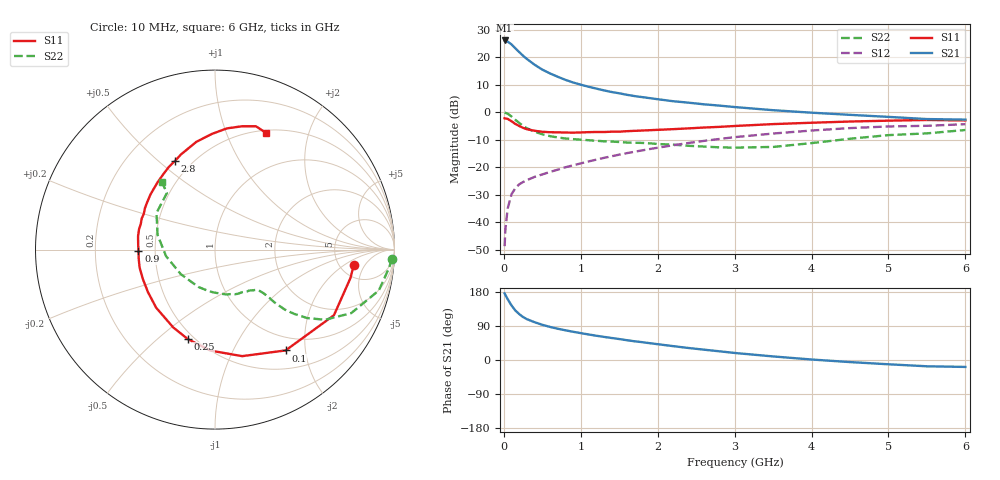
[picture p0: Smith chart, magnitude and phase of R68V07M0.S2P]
! SIEMENS Small Signal Semiconductors
! BFR193
! Si NPN RF Bipolar Junction Transistor in SOT23
! VCE = 8 V  IC = 7 mA
! Common Emitter S-Parameters:  May  1996
# GHz  S  MA  R  50
!  f  S11  S21  S12  S22
! GHz  MAG  ANG  MAG  ANG  MAG  ANG  MAG  ANG
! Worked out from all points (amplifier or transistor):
!   36 points, 10 MHz to 6 GHz, reference 50 ohm
!   highest |S21| = 26.1 dB at 10 MHz (marker M1)
!   |S21| within 3 dB of that: start of sweep to 154.8 MHz
!   unconditionally stable (mu >= 1): 840.8 MHz to 2.029 GHz
!   at 250 MHz: K = 0.52, MSG = 22.9 dB, |S12| = -25.3 dB
!   at 1.4 GHz: K = 1.05, MAG = 10.3 dB, |S12| = -16.0 dB
!   at 6 GHz: K = 0.95, MSG = 0.8 dB, |S12| = -4.3 dB
!   lowest NFmin = 1.20 dB at 450 MHz
!   S11 on the Smith chart (normalised r, x): 10 MHz: 6.75, -2.87; 100 MHz: 0.77, -1.64; 250 MHz: 0.46, -0.63; 900 MHz: 0.40, -0.01; 2.8 GHz: 0.41, +0.57; 6 GHz: 0.53, +1.40
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0.01  0.7776 -6.2  20.12 175.9  0.0037 83.6  0.9866 -2.9
0.02  0.7713 -11.8  20.05 171.6  0.0074 81.0  0.9761 -5.8
0.05  0.7569 -28.9  19.15 160.4  0.0179 75.7  0.9409 -14.0
0.1  0.6858 -55.0  17.06 143.9  0.0325 65.3  0.8375 -25.0
0.15  0.6126 -75.7  14.46 130.5  0.0419 58.9  0.7274 -32.5
0.2  0.5631 -92.7  12.37 121.2  0.0491 54.6  0.6399 -36.6
0.25  0.5205 -107.1  10.63 113.4  0.0542 52.2  0.5671 -39.1
0.3  0.4922 -118.2  9.257 107.8  0.0585 52.0  0.5118 -40.7
0.4  0.4607 -135.4  7.285 99.7  0.0671 52.2  0.4427 -41.6
0.5  0.4423 -147.6  5.951 92.9  0.0743 53.5  0.3978 -41.6
0.6  0.434 -157.8  5.071 87.3  0.0824 55.0  0.3679 -41.9
0.7  0.4318 -166.4  4.414 82.5  0.0906 56.6  0.3487 -42.4
0.9  0.4265 -178.9  3.468 74.5  0.1088 58.3  0.3252 -43.8
1.1  0.4352 170.1  2.909 67.5  0.1278 59.8  0.3109 -46.8
1.3  0.4373 161.1  2.498 61.0  0.1485 60.3  0.2971 -50.2
1.6  0.4532 149.6  2.073 52.2  0.1809 59.8  0.282 -57.3
2.2  0.493 130.4  1.586 36.6  0.2514 56.0  0.2578 -75.8
2.8  0.5427 114.1  1.321 23.0  0.327 49.3  0.2305 -102.8
3.5  0.6095 99.8  1.09 9.4  0.4107 39.2  0.2346 -144.3
4.5  0.6786 84.4  0.897 -5.5  0.5156 23.8  0.3304 165.6
5.5  0.7239 71.7  0.752 -16.6  0.5675 7.4  0.4137 130.4
6  0.7096 66.2  0.735 -18.3  0.607 2.8  0.4762 128.2
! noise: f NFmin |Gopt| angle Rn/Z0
0.45  1.2  0.24  125  0.12
0.9  1.25  0.36  154  0.11
1.8  2  0.55  -156  0.13
